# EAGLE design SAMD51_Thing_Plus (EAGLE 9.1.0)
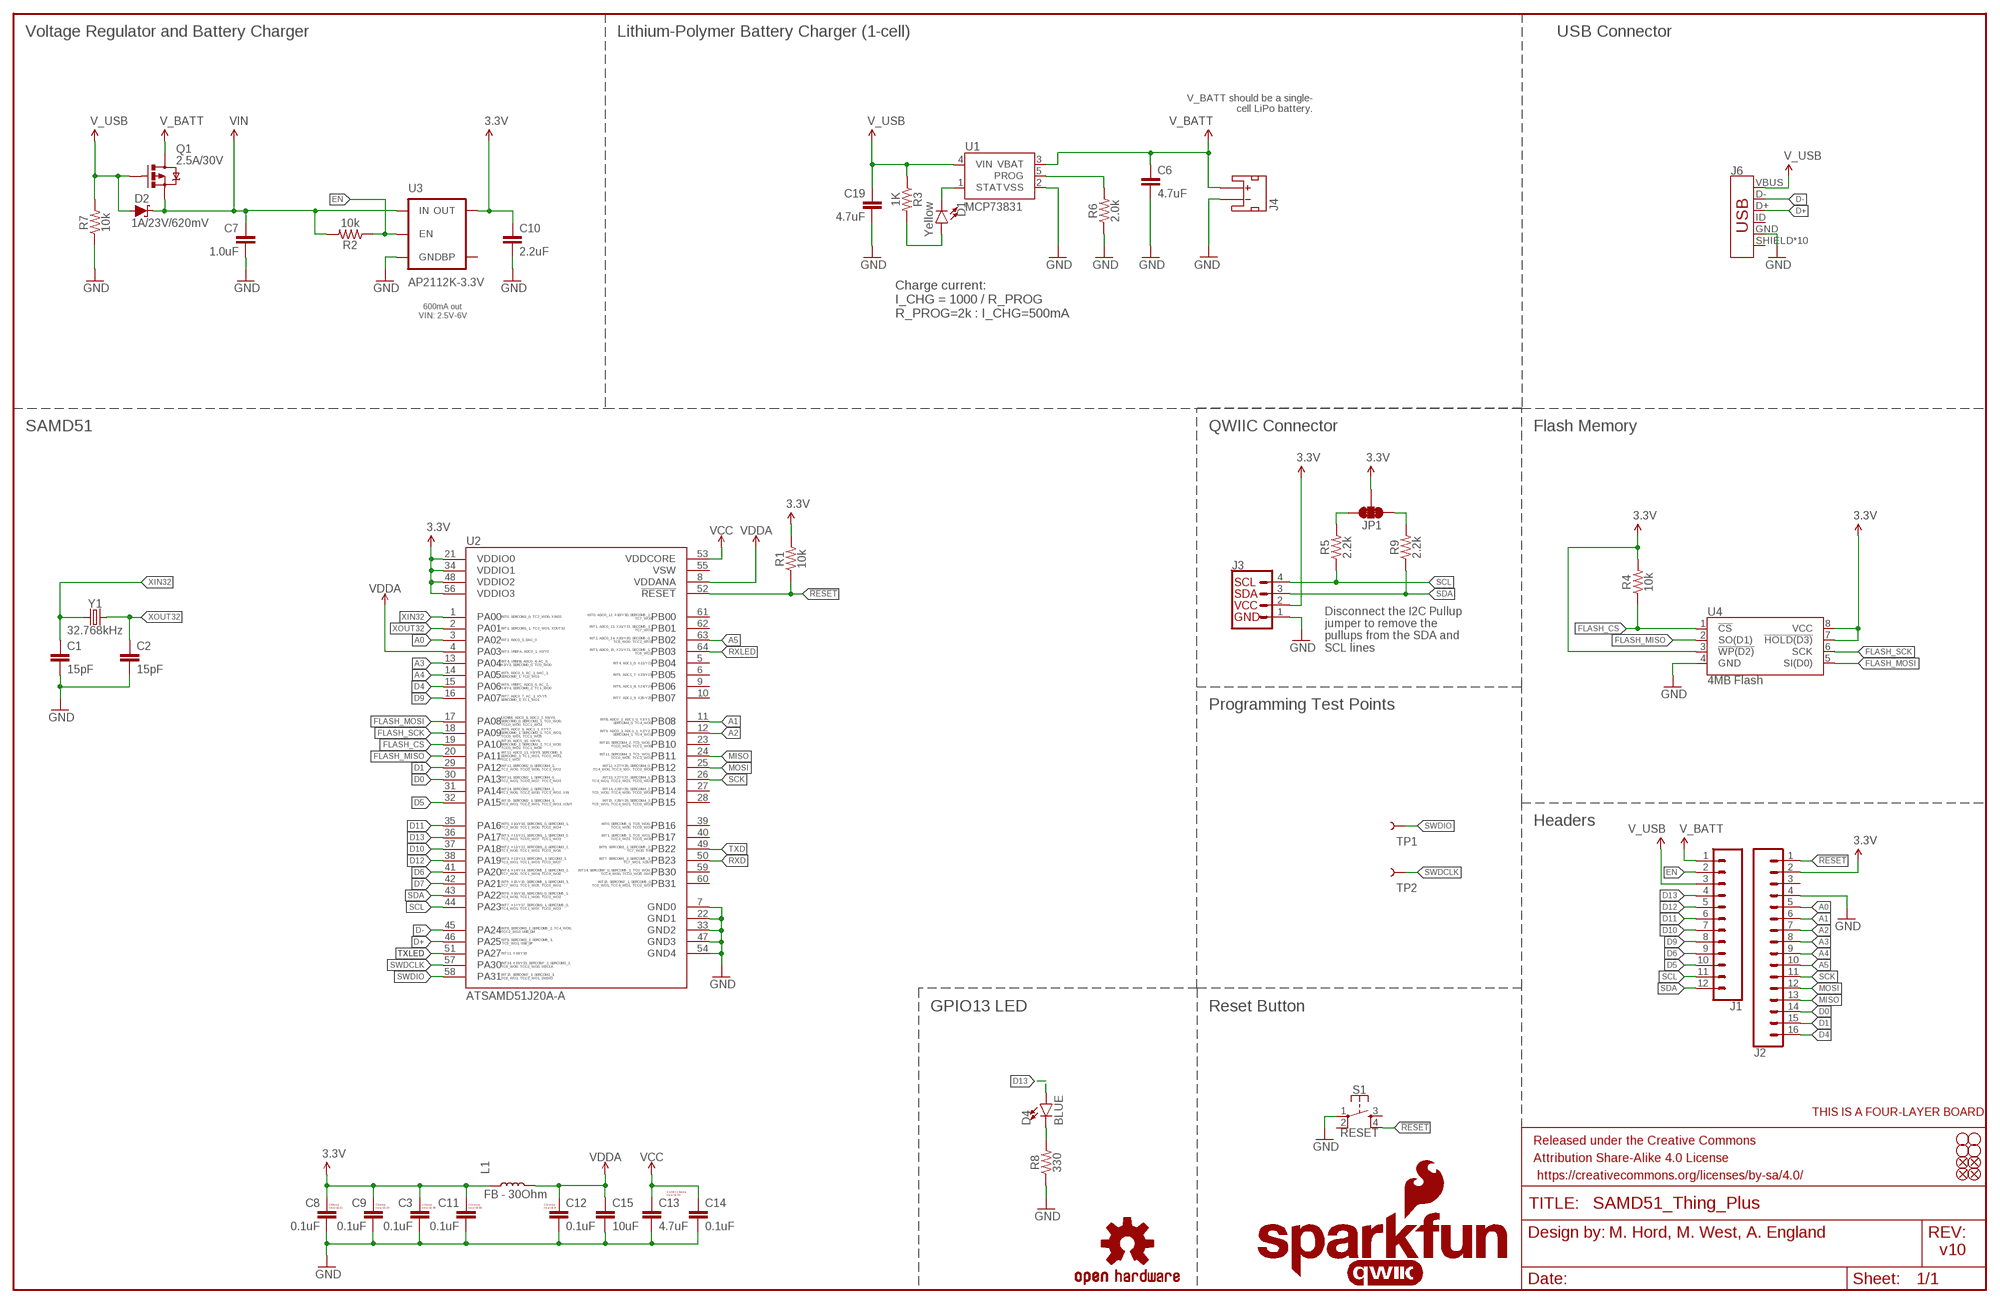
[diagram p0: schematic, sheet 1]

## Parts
C1  15pF  15PF-0402-50V-5%  [0402]
C2  15pF  15PF-0402-50V-5%  [0402]
C3  0.1uF  0.1UF-0402-16V-10%  [0402]
C6  4.7uF  4.7UF-0603-6.3V-(10%)  [0603]
C7  1.0uF  1.0UF-0603-16V-10%-X7R  [0603]
C8  0.1uF  0.1UF-0402-16V-10%  [0402]
C9  0.1uF  0.1UF-0402-16V-10%  [0402]
C10  2.2uF  2.2UF-0603-10V-20%  [0603]
C11  0.1uF  0.1UF-0402-16V-10%  [0402]
C12  0.1uF  0.1UF-0402-16V-10%  [0402]
C13  4.7uF  4.7UF-0603-6.3V-(10%)  [0603]
C14  0.1uF  0.1UF-0402-16V-10%  [0402]
C15  10uF  10UF-0805-10V-10%  [0805]
C19  4.7uF  4.7UF-0603-6.3V-(10%)  [0603]
D1  Yellow  LED-YELLOW0603  [LED-0603]
D2  1A/23V/620mV  DIODE-SCHOTTKY-BAT20J  [SOD-323]
D4  BLUE  LED-BLUE0603  [LED-0603]
FD1  FIDUCIALUFIDUCIAL  [FIDUCIAL-MICRO]
FD2  FIDUCIALUFIDUCIAL  [FIDUCIAL-MICRO]
FD3  FIDUCIALUFIDUCIAL  [FIDUCIAL-MICRO]
FD4  FIDUCIALUFIDUCIAL  [FIDUCIAL-MICRO]
FRAME1  FRAME-LEDGER  [CREATIVE_COMMONS]
H1  STAND-OFF  [STAND-OFF]
H2  STAND-OFF  [STAND-OFF]
H3  STAND-OFF  [STAND-OFF]
H4  STAND-OFF  [STAND-OFF]
J1  CONN_12SM_SQ_NO_SILK  [1X12_SM_SQ_NOSILK]
J2  CONN_161X16_SM_SQ_NOSILK  [1X16_SM_SQ_NOSILK]
J3  QWIIC_CONNECTORJS-1MM  [JST04_1MM_RA]
J4  JST_2MM_MALE  [JST-2-SMD]
J6  AMP FCI 10103594-0001LF  USB_MICRO-B_HALF_PTH_MILL  [USB-MICROB-PTH-MILL]
JP1  JUMPER-SMT_3_2-NC_TRACE_SILK  [SMT-JUMPER_3_2-NC_TRACE_SILK]
L1  FB - 30Ohm  INDUCTORFB-30OHM  [0603]
LOGO1  FOUR_LAYER_WARNING  [FOUR_LAYER_WARNING]
LOGO2  OSHW-LOGOMINI  [OSHW-LOGO-MINI]
LOGO3  SFE_LOGO_NAME_FLAME.1_INCH  [SFE_LOGO_NAME_FLAME_.1]
LOGO4  SFE_LOGO_FLAME.1_INCH  [SFE_LOGO_FLAME_.1]
Q1  2.5A/30V  MOSFET-PCHANNELDMG2307L  [SOT23-3@1]
R1  10k  10KOHM-0603-1/10W-1%  [0603]
R2  10k  10KOHM-0603-1/10W-1%  [0603]
R3  1K  1KOHM-1/10W-1%(0603)  [0603]
R4  10k  10KOHM-0603-1/10W-1%  [0603]
R5  2.2k  2.2KOHM-0603-1/10W-1%  [0603]
R6  2.0k  2.0KOHM1/10W5%(0603)  [0603]
R7  10k  10KOHM-0603-1/10W-1%  [0603]
R8  330  330OHM1/10W1%(0603)  [0603]
R9  2.2k  2.2KOHM-0603-1/10W-1%  [0603]
S1  RESET  MOMENTARY-SWITCH-SPST-2-SMD-4.6X2.8MM  [TACTILE_SWITCH_SMD_4.6X2.8MM]
TP1  TEST-POINTTP_15TH_THRU  [TP_15TH]
TP2  TEST-POINTTP_15TH_THRU  [TP_15TH]
U1  MCP73831  [SOT23-5]
U2  ATSAMD51J20A-A  [TQFP64]
U3  AP2112K-3.3V  V_REG_LDOSMD  [SOT23-5]
U4  4MB Flash  AT25SF041  [SO08]
U$69  QWIIC_LOGO_5MM  [QWIIC_5MM]
Y1  32.768kHz  CRYSTAL-32.768KHZSMD-3.2X1.5  [CRYSTAL-SMD-3.2X1.5MM]

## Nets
3.3V: C3.1 C8.1 C9.1 C10.1 C11.1 J2.2 J3.2 JP1.2 L1.1 R1.2 R4.2 U2.21(VDDIO0) U2.34(VDDIO1) U2.48(VDDIO2) U2.56(VDDIO3) U3.5(OUT) U4.3(!WP(D2)) U4.7(!HOLD(D3)) U4.8(VCC)
!RESET: J2.1 R1.1 S1.4 U2.52(!RESET)
A0: J2.5 U2.3(PA02)
A1: J2.6 U2.11(PB08)
A2: J2.7 U2.12(PB09)
A3: J2.8 U2.13(PA04)
A4: J2.9 U2.14(PA05)
A5: J2.10 U2.63(PB02)
D0: J2.14 U2.30(PA13)
D1: J2.15 U2.29(PA12)
D4: J2.16 U2.15(PA06)
D5: J1.10 U2.32(PA15)
D6: J1.9 U2.41(PA20)
D7: U2.42(PA21)
D9: J1.8 U2.16(PA07)
D10: J1.7 U2.37(PA18)
D11: J1.6 U2.35(PA16)
D12: J1.5 U2.38(PA19)
D13: D4.A J1.4 U2.36(PA17)
D+: J6.D+ U2.46(PA25)
D-: J6.D- U2.45(PA24)
EN: J1.2 R2.1 U3.3(EN)
FLASH_CS: R4.1 U2.19(PA10) U4.1(!CS)
FLASH_MISO: U2.20(PA11) U4.2(SO(D1))
FLASH_MOSI: U2.17(PA08) U4.5(SI(D0))
FLASH_SCK: U2.18(PA09) U4.6(SCK)
GND: C1.2 C2.2 C3.2 C6.2 C7.2 C8.2 C9.2 C10.2 C11.2 C12.2 C13.2 C14.2 C15.2 C19.2 J2.4 J3.1 J4.1(-) J6.GND R6.1 R7.1 R8.1 S1.1 U1.2(VSS) U2.7(GND0) U2.22(GND1) U2.33(GND2) U2.47(GND3) U2.54(GND4) U3.2(GND) U4.4(GND)
MISO: J2.13 U2.24(PB11)
MOSI: J2.12 U2.25(PB12)
N$1: D4.C R8.2
N$2: JP1.3 R5.2
N$3: JP1.1 R9.2
N$9: D1.C U1.1(STAT)
N$14: R6.2 U1.5(PROG)
N$17: D1.A R3.2
RXD: U2.50(PB23)
RXLED: U2.64(PB03)
SCK: J2.11 U2.26(PB13)
SCL: J1.11 J3.4 R5.1 U2.44(PA23)
SDA: J1.12 J3.3 R9.1 U2.43(PA22)
SWDCLK: TP2.P$1 U2.57(PA30)
SWDIO: TP1.P$1 U2.58(PA31)
TXD: U2.49(PB22)
TXLED: U2.51(PA27)
V_BATT: C6.1 J1.1 J4.2(+) Q1.3(D) U1.3(VBAT)
V_USB: C19.1 D2.A J1.3 J6.VBUS Q1.1(G) R3.1 R7.2 U1.4(VIN)
VCC: C13.1 C14.1 U2.53(VDDCORE)
VDDA: C12.1 C15.1 L1.2 U2.4(PA03) U2.8(VDDANA)
VIN: C7.1 D2.C Q1.2(S) R2.2 U3.1(IN)
XIN32: C1.1 U2.1(PA00) Y1.P$1
XOUT32: C2.1 U2.2(PA01) Y1.P$2
Unconnected: J2.3 J4.NC1(PAD1) J4.NC2(PAD2) J6.ID J6.SHIELD J6.SHIELD2(SHIELD) J6.SHIELD3(SHIELD) J6.SHIELD4(SHIELD) J6.SHIELD5(SHIELD) J6.SHIELD6(SHIELD) J6.SHIELD7(SHIELD) J6.SHIELD8(SHIELD) J6.SHIELD9(SHIELD) J6.SHIELD10(SHIELD) S1.2 S1.3 U2.5(PB04) U2.6(PB05) U2.9(PB06) U2.10(PB07) U2.23(PB10) U2.27(PB14) U2.28(PB15) U2.31(PA14) U2.39(PB16) U2.40(PB17) U2.55(VSW) U2.59(PB30) U2.60(PB31) U2.61(PB00) U2.62(PB01) U3.4(BP)

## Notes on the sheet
- Voltage Regulator and Battery Charger | Lithium-Polymer Battery Charger (1-cell)
- USB Connector
- V_BATT should be a single-
  cell LiPo battery.
- Charge current:
  I_CHG = 1000 / R_PROG
  R_PROG=2k : I_CHG=500mA
- 600mA out
  VIN: 2.5V-6V
- SAMD51 | QWIIC Connector | Flash Memory
- Disconnect the I2C Pullup 
  jumper to remove the 
  pullups from the SDA and 
  SCL lines
- Programming Test Points
- Headers
- GPIO13 LED | Reset Button
- C13 & C14 to be
  near U2.53
- C8 to be
  near U2.21
- C9 to be
  near U2.34
- C3 to be
  near U2.48
- C11 to be
  near U2.56
- C12 to be
  near U2.8
- M. Hord, M. West, A. England
- v10

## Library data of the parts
C1 C2 = SparkFun-Capacitors:15PF: 15pF ceramic capacitors; PROD_ID: CAP-13063
C3 C8 C9 C11 C12 C14 = SparkFun-Capacitors:0.1UF: 0.1µF ceramic capacitors; PROD_ID: CAP-12416
C6 C13 C19 = SparkFun-Capacitors:4.7UF: 4.7µF ceramic capacitors; PROD_ID: CAP-08280
C7 = SparkFun-Capacitors:1.0UF: 1µF ceramic capacitors; PROD_ID: CAP-13930
C10 = SparkFun-Capacitors:2.2UF: 2.2µF ceramic capacitors; PROD_ID: CAP-07888
C15 = SparkFun-Capacitors:10UF: 10.0µF ceramic capacitors; PROD_ID: CAP-11330
D1 = SparkFun-LED:LED-YELLOW: Yellow SMD LED; PROD_ID: DIO-09003
D2 = SparkFun-DiscreteSemi:DIODE-SCHOTTKY: Schottky diode; PROD_ID: DIO-11623
D4 = SparkFun-LED:LED-BLUE: Blue SMD LED; PROD_ID: DIO-08575
FD1-FD4 = SparkFun-Aesthetics:FIDUCIAL: Fiducial Alignment Points
FRAME1 = SparkFun-Aesthetics:FRAME-LEDGER: Schematic Frame - Ledger
H1-H4 = SparkFun-Hardware:STAND-OFF: Stand Off
J1 = SparkFun-Connectors:CONN_12: Multi connection point. Often used as Generic Header-pin footprint for 0.1 inch spaced/style header connections On any of the 0.1 inch spaced packages, you can populate with these: Break Away Headers - Straight (PRT-00116) Break Away Male Headers - Right Angle (PRT-00553) Female Headers (PRT-00115)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
J2 = SparkFun-Connectors:CONN_16: Multi connection point. Often used as Generic Header-pin footprint for 0.1 inch spaced/style header connections On any of the 0.1 inch spaced packages, you can populate with these: Break Away Headers - Straight (PRT-00116) Break Away Male Headers - Right Angle (PRT-00553) Female Headers (PRT-00115)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
J3 = SparkFun-Connectors:QWIIC_CONNECTOR: SparkFun I2C Standard Qwiic Connector An SMD 1mm pitch JST connector makes it easy and quick (get it? Qwiic?) to connect I2C devices to each other. The Qwiic system enables fast and solderless connection between popular platforms and various sensors and actuators. We carry 200mm, 100mm, 50mm, and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; PROD_ID: CONN-13694
J4 = SparkFun-Connectors:JST_2MM_MALE: JST 2MM MALE RA CONNECTOR Two pin, compact surface mount connector. Commonly used as a battery input connection point. We really like the solid locking feeling and high current rating on these small connectors. We use these all the time as battery connectors. Mates to single-cell LiPo batteries.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; PROD_ID: CONN-11443; SF_ID: PRT-08612
J6 = SparkFun-Connectors:USB_MICRO-B: USB Type Micro-B Connector Male/female and PTH/SMT variants SparkFun Products: SparkFun microB USB Breakout SparkFun USB microB Plug Breakout SparkFun ESP8266 Thing; PROD_ID: CONN-13711
JP1 = SparkFun-Jumpers:JUMPER-SMT_3_2-NC_TRACE: Normally closed trace jumper (2 of 2 connections) This jumper has a trace between all three pads so they are normally closed (NC). Use a razor knife to open the connection(s). For best results follow the IPC guidelines for cutting traces: Cutout at least 0.063 mm (0.005 in). Remove all loose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
L1 = SparkFun-Coils:INDUCTOR: Inductors; PROD_ID: NDUC-07859
LOGO1 = SparkFun-Aesthetics:FOUR_LAYER_WARNING: Four-Layer Board Warning - tDoc Layer
LOGO2 = SparkFun-Aesthetics:OSHW-LOGO: Open-Source Hardware (OSHW) Logo
LOGO3 = SparkFun-Aesthetics:SFE_LOGO_NAME_FLAME: SparkFun Font Logo w/ Flame
LOGO4 = SparkFun-Aesthetics:SFE_LOGO_FLAME: SparkFun Flame Logo
Q1 = SparkFun-DiscreteSemi:MOSFET-PCHANNEL: Generic PMOSFET IRLML2244 - TRANS-11153 (SOT-23 -20V -4.3A) (1.Gate 2.Source 3.Drain) FQP27P06 - COM-10349 (TO-220 -60V -27A) (1.Gate 2.Source 3.Drain); PROD_ID: TRANS-11308
R1 R2 R4 R7 = SparkFun-Resistors:10KOHM: 10kΩ resistor; PROD_ID: RES-00824
R3 = SparkFun-Resistors:1KOHM-1/10W-1%(0603): RES-07856; PROD_ID: RES-07856
R5 R9 = SparkFun-Resistors:2.2KOHM: 2.2kΩ resistor; PROD_ID: RES-08272
R6 = SparkFun-Resistors:2.0KOHM1/10W5%(0603): RES-08296; PROD_ID: RES-08296
R8 = SparkFun-Resistors:330OHM1/10W1%(0603): RES-00818; PROD_ID: RES-00818
S1 = SparkFun-Switches:MOMENTARY-SWITCH-SPST-2: Momentary Switch (Pushbutton) - SPST - Two Circuits Normally-open (NO) SPST momentary switches (buttons, pushbuttons). Schematic symbol includes two switch circuits. Variants SMD-4.6MMX2.8MM - 4.60mm x 2.80mm Tactile Momentary Button Switch - Used on SparkFun SAMD21 Mini Breakout SMD-5.2MM - Mini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; PROD_ID: SWCH-13065
TP1 TP2 = SparkFun-Connectors:TEST-POINT: SparkFun Test Points
U1 = SparkFun-PowerIC:MCP73831: Miniature single cell, fully integrated Li-Ion, Li-polymer charge management controller http://ww1.microchip.com/downloads/en/DeviceDoc/20001984g.pdf IC-09995; PROD_ID: IC-09995
U2 = SparkFun-IC-Microcontroller:ATSAMD51J20A-A; PROD_ID: IC-13952
U3 = SparkFun-PowerIC:V_REG_LDO: Voltage Regulator LDO Standard 150mA LDO voltage regulator in SOT-23 layout. Micrel part MIC5205. BP (by-pass) pin is used to lower output noise with 470pF cap.; PROD_ID: VREG-12457
U4 = SparkFun-IC-Memory:AT25SF041: AT25SF041 4Mb Serial Flash Memory 104MHz, SPI, 8-SOIC Datasheet SparkFun Products: SparkFun ESP8266 Thing SparkFun ESP8266 Thing - Dev Board; PROD_ID: IC-12455
U$69 = SparkFun-Aesthetics:QWIIC_LOGO: Qwiic Logos for placement on schematic and PCB. The 5.5mm silk logo is best for placing next to Qwiic connector.
Y1 = SparkFun-Clocks:CRYSTAL-32.768KHZ: 32.768kHz Crystal; PROD_ID: XTAL-13062

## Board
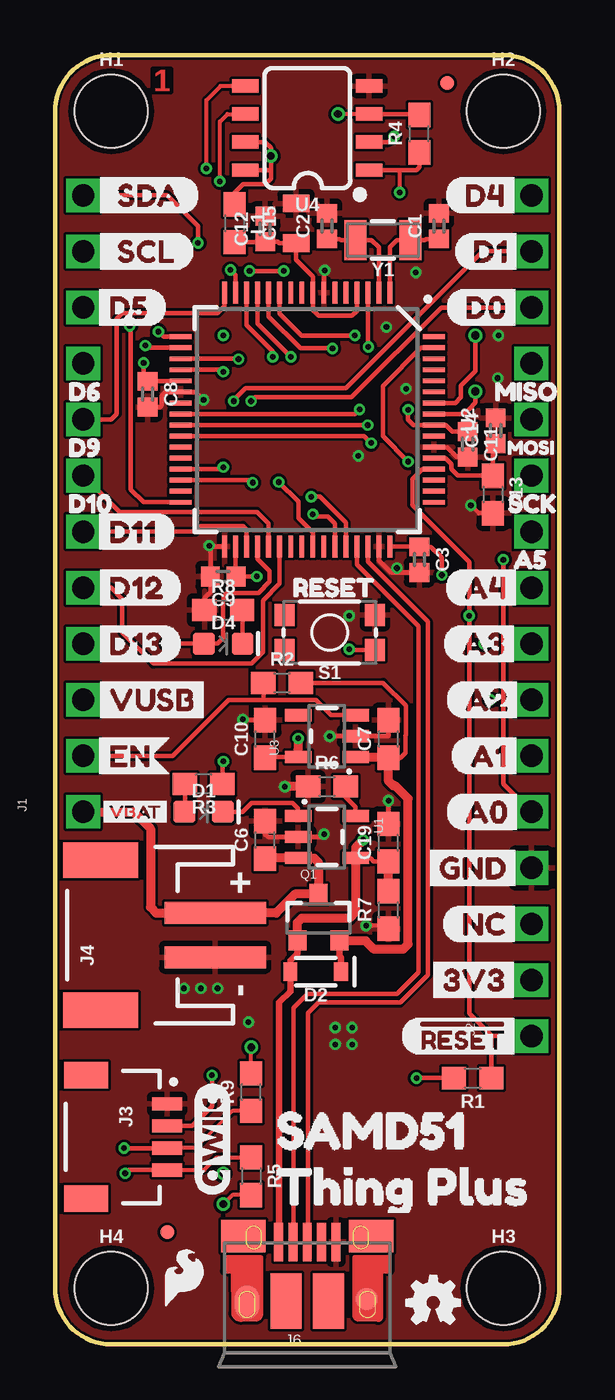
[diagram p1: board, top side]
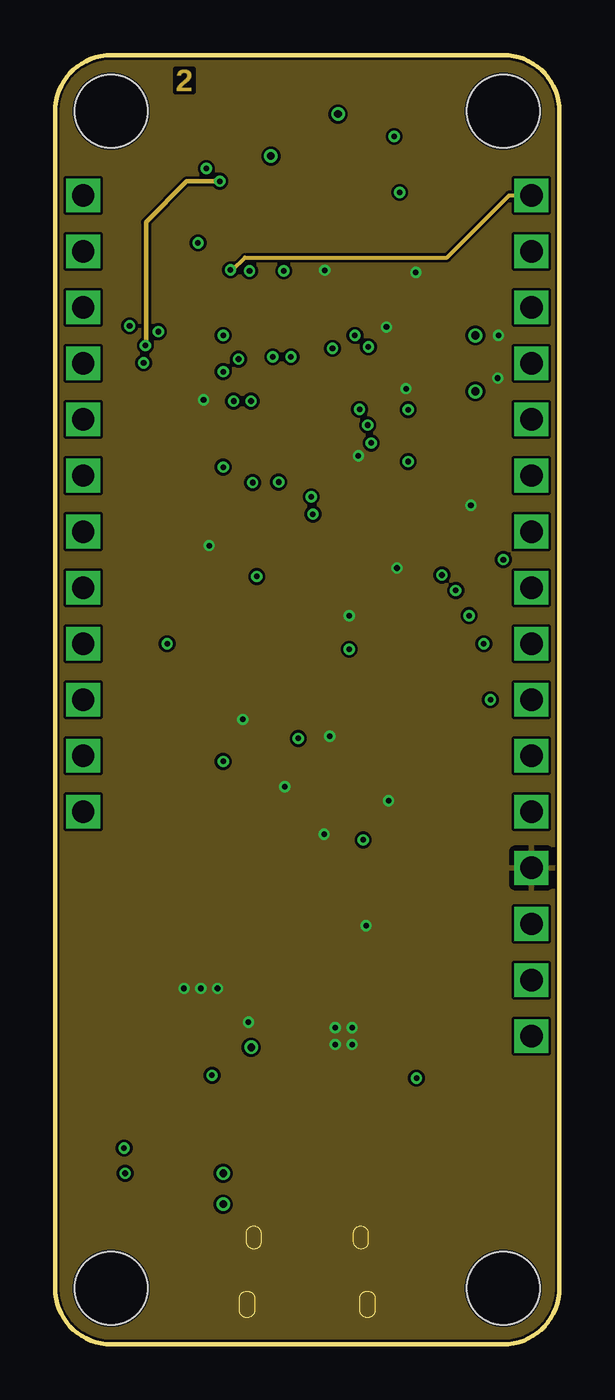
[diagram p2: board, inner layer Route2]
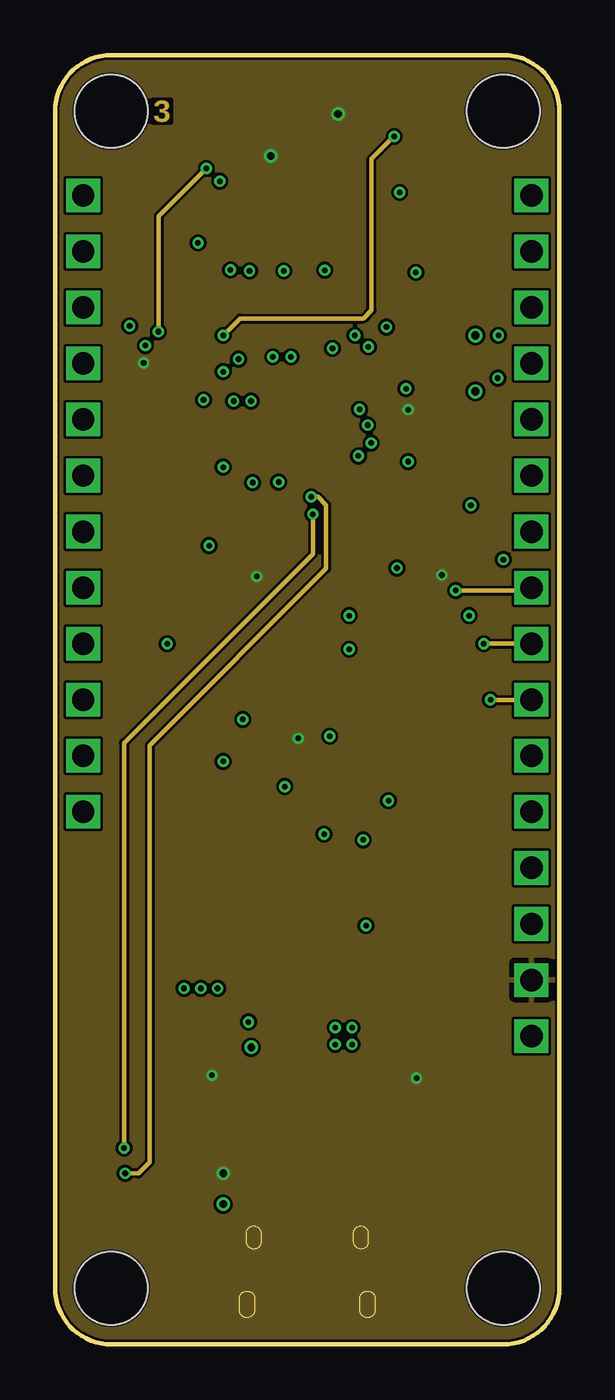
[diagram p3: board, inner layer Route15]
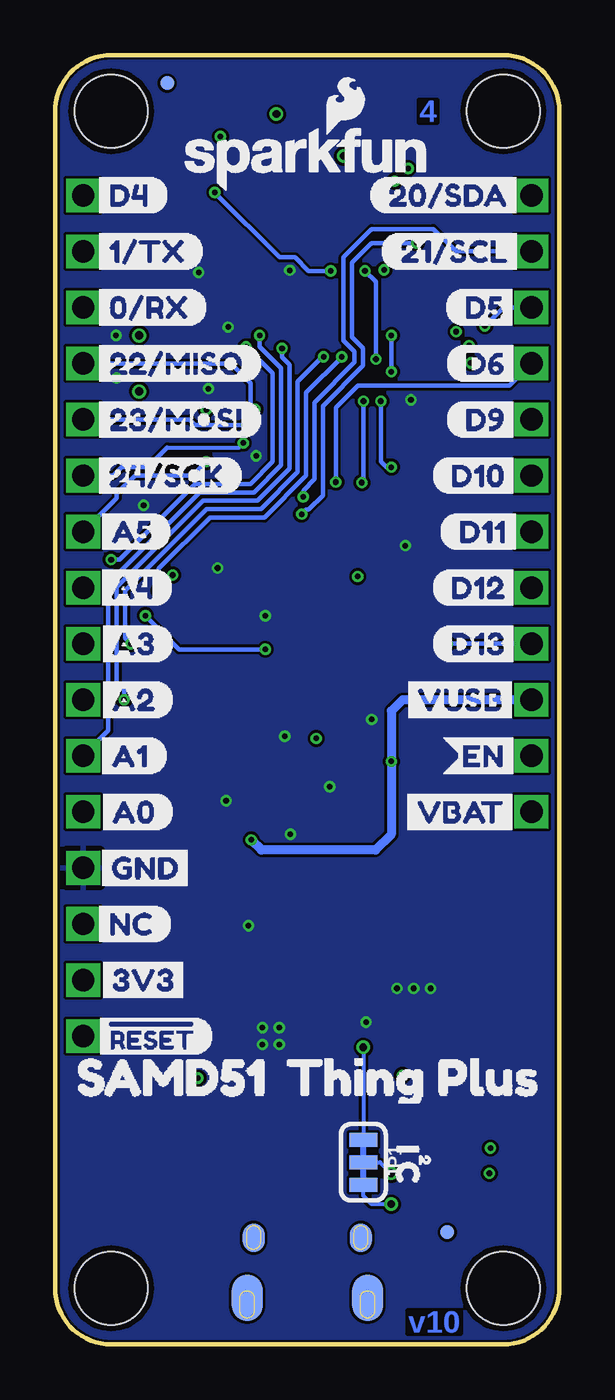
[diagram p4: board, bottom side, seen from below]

Size 22.86 x 58.42 mm. Coordinates in mm from the lower left corner, seen from the top.
Outline: 2.54,58.42 20.32,58.42 arc-90 22.86,55.88 22.86,2.54 arc-90 20.32,0 2.54,0 arc-90 0,2.54 0,55.88 arc-90 2.54,58.42
Copper layers (1*2*15*16): Top 0.035559375mm / dielectric 0.47751875mm / Route2 0.035559375mm / dielectric 0.47751875mm / Route15 0.035559375mm / dielectric 0.47751875mm / Bottom 0.035559375mm
Design rules "SparkFun-4-layer-FAB-LIMIT": minimum track width 4mil, minimum drill 6mil, track to track 5mil, track to pad 5mil, pad to pad 5mil, via to via 5mil, smd to smd 5mil, copper to edge 4mil, drill to drill 4mil, minimum pad ring 5mil, minimum via ring 5mil, stop-mask expansion 4mil, vias tented up to drill 25mil, thermal gap 10mil

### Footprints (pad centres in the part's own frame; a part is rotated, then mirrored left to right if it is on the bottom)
0402 = smd 0.85 x 0.9: 1 -0.58,0; 2 0.58,0
0603 = smd 1.1 x 1: 1 -0.85,0; 2 0.85,0
0805 = smd 0.8 x 1.2: 1 -0.9,0; 2 0.9,0
LED-0603 = smd 1 x 1: A -0.877,0; C 0.877,0
SOD-323 = smd 0.63 x 0.83: A 1.15,0; C -1.15,0
FIDUCIAL-MICRO = smd 0.635 x 0.635: 1 0,0
STAND-OFF = hole 3.302: 0,0
1X12_SM_SQ_NOSILK = drill 1.016 pad 1.27 square: 1 0,0; 2 2.54,0; 3 5.08,0; 4 7.62,0; 5 10.16,0; 6 12.7,0; 7 15.24,0; 8 17.78,0; 9 20.32,0; 10 22.86,0; 11 25.4,0; 12 27.94,0
1X16_SM_SQ_NOSILK = drill 1.016 pad 1.27 square: 1 0,0; 2 2.54,0; 3 5.08,0; 4 7.62,0; 5 10.16,0; 6 12.7,0; 7 15.24,0; 8 17.78,0; 9 20.32,0; 10 22.86,0; 11 25.4,0; 12 27.94,0; 13 30.48,0; 14 33.02,0; 15 35.56,0; 16 38.1,0
JST04_1MM_RA = smd 0.6 x 1.35: 1 -1.5,0; 2 -0.5,0; 3 0.5,0; 4 1.5,0 | smd 1.2 x 2: NC1 2.8,-3.675; NC2 -2.8,-3.675
JST-2-SMD = smd 1 x 4.6: 1 -1,-3.7; 2 1,-3.7 | smd 1.6 x 3.4: NC1 -3.4,1.5; NC2 3.4,1.5
USB-MICROB-PTH-MILL = smd 0.4 x 1.75: D+ 0,0; D- -0.65,0; GND 1.3,0; ID 0.65,0; VBUS -1.3,0 | smd 2 x 1.46: SHIELD -2.9,0.275; SHIELD2 2.9,0.275 | smd 1.425 x 2.5: SHIELD3 -0.963,-2.675; SHIELD4 0.963,-2.675 | smd 1.4 x 2.1 bottom: SHIELD5 -2.731,-2.531; SHIELD7 2.729,-2.531 | smd 1 x 1: SHIELD6 2.7,-2.575 | smd 1.1 x 1.5: SHIELD8 -2.731,-2.731 | smd 1 x 1.3 bottom: SHIELD9 -2.43,0.195; SHIELD10 2.43,0.195
SMT-JUMPER_3_2-NC_TRACE_SILK = smd 0.635 x 1.27: 1 -1.016,0; 2 0,0; 3 1.016,0
SOT23-3@1 = smd 0.8 x 0.9: 1 -0.95,-1; 2 0.95,-1; 3 0,1.1
TACTILE_SWITCH_SMD_4.6X2.8MM = smd 0.9 x 1: 1 -2.05,-0.8; 2 2.05,-0.8; 3 2.05,0.8; 4 -2.05,0.8
TP_15TH = drill 0.381 pad 0.61: P$1 0,0
SOT23-5 = smd 0.55 x 1.2: 1 -0.95,-1.3; 2 0,-1.3; 3 0.95,-1.3; 4 0.95,1.3; 5 -0.95,1.3
TQFP64 = smd 0.22 x 1: 1 -3.75,-5.75; 2 -3.25,-5.75; 3 -2.75,-5.75; 4 -2.25,-5.75; 5 -1.75,-5.75; 6 -1.25,-5.75; 7 -0.75,-5.75; 8 -0.25,-5.75; 9 0.25,-5.75; 10 0.75,-5.75; 11 1.25,-5.75; 12 1.75,-5.75; 13 2.25,-5.75; 14 2.75,-5.75; 15 3.25,-5.75; 16 3.75,-5.75; 33 3.75,5.75; 34 3.25,5.75; 35 2.75,5.75; 36 2.25,5.75; 37 1.75,5.75; 38 1.25,5.75; 39 0.75,5.75; 40 0.25,5.75; 41 -0.25,5.75; 42 -0.75,5.75; 43 -1.25,5.75; 44 -1.75,5.75; 45 -2.25,5.75; 46 -2.75,5.75; 47 -3.25,5.75; 48 -3.75,5.75 | smd 1 x 0.22: 17 5.75,-3.75; 18 5.75,-3.25; 19 5.75,-2.75; 20 5.75,-2.25; 21 5.75,-1.75; 22 5.75,-1.25; 23 5.75,-0.75; 24 5.75,-0.25; 25 5.75,0.25; 26 5.75,0.75; 27 5.75,1.25; 28 5.75,1.75; 29 5.75,2.25; 30 5.75,2.75; 31 5.75,3.25; 32 5.75,3.75; 49 -5.75,3.75; 50 -5.75,3.25; 51 -5.75,2.75; 52 -5.75,2.25; 53 -5.75,1.75; 54 -5.75,1.25; 55 -5.75,0.75; 56 -5.75,0.25; 57 -5.75,-0.25; 58 -5.75,-0.75; 59 -5.75,-1.25; 60 -5.75,-1.75; 61 -5.75,-2.25; 62 -5.75,-2.75; 63 -5.75,-3.25; 64 -5.75,-3.75
SO08 = smd 0.6 x 1.2: 1 -1.905,-2.8; 2 -0.635,-2.8; 3 0.635,-2.8; 4 1.905,-2.8; 5 1.905,2.8; 6 0.635,2.8; 7 -0.635,2.8; 8 -1.905,2.8
CRYSTAL-SMD-3.2X1.5MM = smd 1 x 1.8: P$1 -1.25,0; P$2 1.25,0

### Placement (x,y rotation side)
C1  17.4,50.67 90 top
C2  12.32,50.67 90 top
C3  16.51,35.56 270 top
C6  9.53,22.86 90 top
C7  15.11,27.43 90 top
C8  4.19,43.05 270 top
C9  7.62,34.8 180 top
C10  9.53,27.43 90 top
C11  18.7,40.79 270 top
C12  9.53,50.55 90 top
C13  19.84,38.51 270 top
C14  19.97,41.4 90 top
C15  10.92,50.8 90 top
C19  15.11,22.73 90 top
D1  6.73,24.13 0 top
D2  11.81,16.89 180 top
D4  7.62,31.75 0 top
FD1  5.08,5.08 0 top
FD2  17.78,57.15 0 top
FD3  5.08,5.08 0 bottom
FD4  17.78,57.15 0 bottom
FRAME1  not placed on the board
H1  2.54,55.88 0 top
H2  20.32,55.88 0 top
H3  20.32,2.54 0 top
H4  2.54,2.54 0 top
J1  1.27,24.13 90 top
J2  21.59,13.97 90 top
J3  5.08,9.4 270 top
J4  3.56,18.54 90 top
J6  11.43,4.64 0 top
JP1  8.89,8.26 270 bottom
L1  8.13,50.8 270 top
LOGO1  not placed on the board
LOGO2  17.14,1.91 0 top
LOGO3  11.43,53.72 0 bottom
LOGO4  5.84,3.05 0 top
Q1  11.94,19.3 0 top
R1  18.92,12.06 180 top
R2  10.29,29.97 0 top
R3  6.73,25.4 180 top
R4  16.51,54.86 90 top
R5  8.89,7.62 270 top
R6  12.32,25.27 0 top
R7  15.11,19.68 90 top
R8  7.62,33.27 0 top
R9  8.89,11.43 90 top
S1  12.45,32.26 180 top
TP1  19.05,45.72 0 top
TP2  19.05,43.18 0 top
U1  12.32,22.99 270 top
U2  11.43,41.91 180 top
U3  12.32,27.56 90 top
U4  11.43,55.12 90 top
U$4  [RESET27]  10.03,34.29 0 top
U$5  [#RESET15]  21.46,13.97 0 bottom
U$6  [#RESET0]  15.49,13.97 0 top
U$7  [3V32]  16.64,16.51 0 top
U$8  [A04]  17.65,24.13 0 top
U$9  [A15]  17.91,26.67 0 top
U$10  [A26]  17.65,29.21 0 top
U$11  [A37]  17.53,31.75 0 top
U$12  [A48]  17.65,34.29 0 top
U$13  [A523]  20.07,35.56 0 top
U$14  [SCK24]  19.81,38.1 0 top
U$15  [3V33]  21.21,16.51 0 bottom
U$16  [MISO26]  19.18,43.18 0 top
U$17  [D09]  17.65,46.99 0 top
U$18  [D110]  18.03,49.53 0 top
U$19  [D411]  17.65,52.07 0 top
U$20  [GND3]  16.51,21.59 0 top
U$21  [GND0]  21.21,21.59 0 bottom
U$22  [EN0]  1.52,26.67 0 top
U$23  [VUSB2]  1.52,29.21 0 top
U$24  [D1312]  1.52,31.75 0 top
U$25  [D120]  1.52,34.29 0 top
U$26  [D1113]  1.52,36.83 0 top
U$27  [A014]  21.21,24.13 0 bottom
U$28  [A113]  21.21,26.67 0 bottom
U$29  [D515]  1.52,46.99 0 top
U$30  [_SCL16]  1.52,49.53 0 top
U$31  [ORDERING_INSTRUCTIONS]  not placed on the board
U$32  [_SDA17]  1.52,52.07 0 top
U$33  [D63]  -0.13,43.18 0 top
U$34  [D92]  -0.13,40.64 0 top
U$35  [MOSI0]  19.94,40.64 0 top
U$36  [VBAT1]  1.91,24.13 0 top
U$37  [A212]  21.21,29.21 0 bottom
U$38  [A311]  21.21,31.75 0 bottom
U$39  [A410]  21.21,34.29 0 bottom
U$40  [A59]  21.21,36.83 0 bottom
U$41  [21#SCL1]  8.13,49.53 0 bottom
U$42  [22#MISO4]  21.34,44.45 0 bottom
U$43  [23#MOSI3]  21.34,41.91 0 bottom
U$44  [1#TX1]  21.34,49.53 0 bottom
U$46  [D41]  21.34,52.07 0 bottom
U$47  [24#SCK2]  21.34,39.37 0 bottom
U$48  [0#RX0]  21.34,46.99 0 bottom
U$49  [D518]  5.21,46.99 0 bottom
U$50  [D619]  5.21,44.45 0 bottom
U$51  [D920]  5.21,41.91 0 bottom
U$52  [D1122]  5.46,36.83 0 bottom
U$53  [D1021]  5.84,39.37 0 bottom
U$54  [D1223]  5.84,34.29 0 bottom
U$55  [D1324]  5.84,31.75 0 bottom
U$56  [VUSB1]  7.37,29.21 0 bottom
U$57  [EN25]  5.33,26.67 0 bottom
U$58  [VBAT2]  7.37,24.13 0 bottom
U$59  [D100]  -0.13,38.1 0 top
U$60  [NC0]  17.53,19.05 0 top
U$61  [NC1]  21.34,19.05 0 bottom
U$62  [20#SDA0]  8.64,52.07 0 bottom
U$63  [SAMD510]  8.89,9.53 0 top
U$64  [THING_PLUS1]  8.89,6.99 0 top
U$65  [SAMD510]  23.02,11.94 0 bottom
U$66  [THING_PLUS1]  13.49,11.94 0 bottom
U$67  [I_C0]  6.86,9.91 270 bottom
U$68  [21]  6.1,9.02 270 bottom
U$69  7.11,9.27 90 top
Y1  14.86,50.04 180 top

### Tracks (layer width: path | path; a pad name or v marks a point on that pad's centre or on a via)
3.3V  (via drill 0.25, 0.35)
  Top 0.178: U4.3 12.89,55.75 v12.83,55.75
  Top 0.203: U2.48 16.49,36.16 C3.1 17.04,36.14 17.53,35.65 v17.53,34.86 | U2.34 8.18,34.82 C9.1 v9.14,34.8 | U2.21 4.22,43.66 C8.1 4.01,43.81 v4.01,44.48 | U3.5 9.55,26.61 C10.1 | R1.2 v16.38,12.06 | U4.3 16.47,55.75 R4.2 | C11.1 18.01,41.37 17.71,41.66 U2.56 16.25,41.66 16,41.91 v16,42.35 | L1.1 8.13,52.2 8.51,52.58 9.53,52.58 9.78,52.83 9.78,53.21 | U4.7 9.53,54.48 9.78,54.23 v9.78,53.85 9.78,53.21 | U4.8 9.78,53.21 | v7.11,12.19 7.11,10.79 6.21,9.9 J3.2
  Top 0.406: U3.5 11.02,26.99 v11.02,27.46
  Bottom 0.178: JP1.2 8.13,8.26 v7.62,7.75
  pour Route15: 0,58.42 22.86,58.42 22.86,0 0,0
!RESET  (via drill 0.25)
  Top 0.203: S1.4 13.37,31.46 | U2.52 16.64,39.66 16.19,39.21 16.19,38.1 16.19,38.04 18.77,35.46 v18.77,33.02 18.77,15 19.77,14 19.77,13.97 | 19.77,13.97 R1.1 | J2.1 19.77,13.97
  Top 0.254: 13.37,31.46 v13.34,31.5
  Bottom 0.203: v13.34,31.5 17.25,31.5 v18.77,33.02
A0  (via drill 0.25)
  Top 0.203: v20.32,35.56 20.32,25.4 J2.5 | U2.3 14.18,45.22 v14.2,45.2
  Bottom 0.203: 13.01,44.01 13.01,39.99 14.01,38.99 16.51,38.99 19.94,35.56 v20.32,35.56 | 13.01,44.01 | 13.01,44.01 v14.2,45.2
A1  (via drill 0.25)
  Top 0.203: U2.11 10.18,46.72 11.18,45.72 v13.59,45.72
  Bottom 0.203: v13.59,45.72 13.59,45.21 12.62,44.25 12.62,39.83 13.85,38.61 16.32,38.61 20.45,34.48 20.45,27.81 J2.6
A2  (via drill 0.25)
  Top 0.203: U2.12 9.68,46.58 11.12,45.14 v12.57,45.14
  Route15 0.203: v19.74,29.21 J2.7
  Bottom 0.203: v12.57,45.14 12.57,44.74 12.24,44.41 12.24,39.68 13.69,38.23 16.16,38.23 20.07,34.32 20.07,29.97 19.74,29.64 v19.74,29.21
A3  (via drill 0.25)
  Top 0.203: U2.13 9.18,46.26 v10.69,44.74
  Route15 0.203: v19.43,31.75 J2.8
  Bottom 0.203: v10.69,44.74 10.76,44.74 11.86,43.64 11.86,39.52 13.53,37.85 16,37.85 19.68,34.16 19.68,32 v19.43,31.75
A4  (via drill 0.25)
  Top 0.203: U2.14 8.68,46.18 9.86,45 v9.86,44.74
  Route15 0.203: v18.16,34.16 21.46,34.16 J2.9
  Bottom 0.203: v9.86,44.74 11.48,43.13 11.48,39.36 13.38,37.47 15.85,37.47 18.16,35.15 v18.16,34.16
A5  (via drill 0.25)
  Top 0.203: U2.63 16.59,45.16 14.86,43.43 14.86,41.15 v16,40.01
  Bottom 0.203: v16,40.01 16.64,39.37 19.24,39.37 20.07,38.54 20.07,38.35 J2.10
D0  (via drill 0.25)
  Top 0.203: J2.14 17.5,46.99 13.44,42.93 9.06,42.93 v8.88,42.74 | v8.95,39.05 8.84,39.16 U2.30
  Bottom 0.203: v8.88,42.74 8.88,39.12 v8.95,39.05
D1  (via drill 0.25)
  Top 0.203: v8.09,42.74 8.09,42.78 8.64,43.33 13.19,43.33 19.39,49.53 J2.15 | v7.62,39.75 7.53,39.66 U2.29
  Bottom 0.203: v8.09,42.74 8.09,40.01 7.84,39.75 v7.62,39.75
D4  (via drill 0.25)
  Top 0.203: U2.15 8.18,48.46 v7.95,48.69
  Route2 0.178: v7.95,48.69 8.05,48.69 8.61,49.24 17.76,49.24 20.59,52.07 J2.16
D5  (via drill 0.25)
  Top 0.203: U2.32 4,38.16 3.43,38.73 3.43,44.45 3.43,46.1 v3.38,46.15
  Bottom 0.203: v3.38,46.15 2.54,46.99 J1.10
D6  (via drill 0.25)
  Top 0.203: v10.13,39.08 11.03,38.19 11.03,37.45 11.68,36.8 U2.41
  Bottom 0.203: v10.13,39.08 10.13,42.44 9.12,43.45 2.27,43.45 J1.9
D9
  Top 0.203: U2.16 7.68,47.05 7.37,46.74 3.05,46.74 2.79,46.48 2.79,42.16 2.54,41.91 J1.8
D10
  Top 0.203: U2.37 9.68,37.18 9.14,37.72 2.92,37.72 J1.7
D11
  Top 0.203: U2.35 8.68,36.91 8.51,37.08 6.6,37.08 6.35,36.83 J1.6
D12
  Top 0.203: J1.5 2.54,34.29 3.05,33.78 3.05,32.26 4.46,30.84 8.9,30.84 9.43,31.37 9.43,33.72 10.18,34.47 U2.38
D13  (via drill 0.25)
  Top 0.203: U2.36 9.18,35.59 9.73,35.04 9.73,34.56 9.23,34.05 7.8,34.05 7.64,33.89 7.64,33.68 7.62,33.66 7.62,32 7.37,31.75 D4.A 5.46,31.75 v5.08,31.75
  Bottom 0.203: v5.08,31.75 J1.4
D+
  Top 0.203: J6.D+ 11.46,4.66 11.46,15.01 11.94,15.49 15.65,15.49 16.89,16.73 16.89,32.77 14.18,35.48 U2.46
D-
  Top 0.203: U2.45 13.68,35.34 14.61,34.42 16.48,32.55 16.48,16.86 15.49,15.88 11.43,15.88 10.81,15.25 10.81,4.66 J6.D-
EN
  Top 0.203: J1.2 5.33,26.67 7.86,29.19 9.4,29.19 | U3.3 12.51,28.51 11.83,29.19 9.4,29.19 | R2.1 9.44,29.23 9.4,29.19
FLASH_CS  (via drill 0.25)
  Top 0.178: v15.62,52.2 15.62,53.15 15.56,53.21
  Top 0.203: 15.56,53.21 15.24,53.21 | 15.24,53.21 U4.1 | v10.36,48.64 v8.81,48.64 | U2.19 8.3,44.66 v8.31,44.64 | 15.24,53.21 16.38,53.21 16.51,53.34 R4.1
  Bottom 0.203: v15.62,52.2 12.68,49.26 11.98,49.26 11.37,48.64 v10.36,48.64 | v8.81,48.64 8.31,48.15 v8.31,44.64
FLASH_MISO  (via drill 0.25)
  Top 0.203: 7.54,44.16 v7.62,44.08 7.54,44.16 | U4.2 15.11,54.48 v15.37,54.74 | 7.54,44.16 U2.20
  Route15 0.203: v7.62,45.72 8.38,46.48 13.97,46.48 14.35,46.86 14.35,53.72 v15.37,54.74
  Bottom 0.203: v7.62,44.08 v7.62,45.72
FLASH_MOSI  (via drill 0.25)
  Top 0.178: U4.5 7.49,57.02 6.86,56.39 v6.86,53.29
  Top 0.203: v4.68,45.89 4.91,45.66 U2.17
  Route15 0.203: v6.86,53.29 4.7,51.13 4.7,45.91 v4.68,45.89
FLASH_SCK  (via drill 0.25)
  Top 0.178: v7.47,52.7 7.47,55.41 7.81,55.75 U4.6
  Top 0.203: U2.18 4.19,45.16 v4.09,45.26
  Route2 0.203: v7.47,52.7 5.97,52.7 4.12,50.85 4.12,45.24 v4.09,45.26
GND  (via drill 0.25)
  Top 0.178: C13.2 19.21,37.66 v18.85,38.02
  Top 0.203: C6.2 9.53,23.11 9.65,22.99 U1.2 12.06,22.99 v12.19,23.11 | C19.2 v15.11,24.64 | v12.45,27.56 U3.2 15.11,27.56 C7.2 | C10.2 8.55,28.28 v8.51,28.32 | R8.1 6.77,33.82 7.04,34.09 C9.2 7.04,36.14 v6.99,36.2 7.02,36.16 U2.33 | R7.1 14.97,18.97 v14.1,18.97 | v6.73,42.8 6.37,43.16 U2.22 4.99,43.16 4.83,43 4.83,42.55 4.75,42.47 C8.2 | U2.7 12.18,48.63 v12.22,48.67 | U2.54 17.2,40.64 17.78,40.64 18.21,40.21 C11.2 | U2.47 14.68,35.52 15.22,34.98 C3.2
  Top 0.406: R6.1 v10.41,25.27
  other vias: 20.07,43.78 15.49,35.18 13.34,33.02 12.7,13.59 12.7,14.35 13.46,14.35 13.46,13.59 5.84,16.13 6.6,16.13 7.37,16.13 8.76,14.61 16.35,48.58 13.75,40.26 20.1,45.72 15.02,46.1 15.91,43.31
  pour Top: 0,58.42 22.86,58.42 22.86,0 0,0
  pour Route2: 0,58.42 22.86,58.42 22.86,0 0,0
  pour Bottom: 0,58.42 22.86,58.42 22.86,0 0,0
MISO  (via drill 0.25)
  Top 0.203: U2.24 13.59,42.16 v13.8,42.37
  Bottom 0.203: v13.8,42.37 14,42.57 14,43.57 14.88,44.45 J2.13
MOSI  (via drill 0.25)
  Top 0.203: U2.25 v14.17,41.66
  Bottom 0.203: J2.12 16.76,41.91 16.51,41.66 v14.17,41.66
N$1
  Top 0.203: R8.2 8.5,33.25 D4.C
N$2  (via drill 0.35)
  Top 0.178: R5.2 8.04,6.77 v7.62,6.35
  Bottom 0.178: v7.62,6.35 8.51,6.35 8.89,6.73 JP1.3
N$3  (via drill 0.35)
  Top 0.178: R9.2 v8.89,13.46
  Bottom 0.178: v8.89,13.46 JP1.1
N$9
  Top 0.203: D1.C 8.5,24.13 8.91,24.54 10.77,24.54 11.02,24.29 U1.1
N$14
  Top 0.203: U1.5 13.62,24.35 13.17,24.8 R6.2
N$17
  Top 0.203: R3.2 5.88,24.16 D1.A
SCK  (via drill 0.25)
  Top 0.203: v14.33,40.84 14.01,41.16 U2.26
  Bottom 0.178: 17.78,40.64 14.53,40.64 v14.33,40.84
  Bottom 0.203: J2.11 20.22,39.37 19.84,39.75 18.67,39.75 17.78,40.64
SCL  (via drill 0.25)
  Top 0.178: R5.1 7.33,8.47 6.75,7.9 J3.4
  Top 0.203: U2.44 13.18,37.24 12.01,38.41 v11.61,38.41 | J3.4 3.33,7.9 v3.17,7.75
  Route15 0.203: v11.61,38.41 11.92,38.41 12.29,38.04 12.29,35.15 4.29,27.15 4.29,8.26 3.78,7.75 v3.17,7.75
  Bottom 0.203: v11.61,38.41 11.61,38.69 11.1,39.2 11.1,42.68 9.28,44.5 9.28,44.99 9.78,45.48 9.78,49.28 8.51,50.55 5.71,50.55 4.7,49.53 J1.11
SDA  (via drill 0.25)
  Top 0.152: 8.04,10.58 6.36,8.9 6.34,8.9
  Top 0.178: 6.34,8.9 J3.3 | R9.1 8.04,10.58
  Top 0.203: U2.43 12.68,37.2 12.37,37.51 11.79,37.51 v11.68,37.62 | J3.3 v3.12,8.89 | v6.48,49.91 6.48,50.67 5.08,52.07 J1.12
  Route15 0.203: v11.68,37.62 11.68,35.81 3.12,27.25 v3.12,8.89
  Bottom 0.203: v11.68,37.62 11.48,37.82 11.37,37.82 10.72,38.47 10.72,42.52 8.9,44.34 8.9,45.14 9.4,45.64 9.4,49.02 8.51,49.91 v6.48,49.91
SWDCLK
  Top 0.203: U2.57 18.54,42.16 18.91,42.53 18.91,42.54 19.05,42.68 TP2.P$1
SWDIO
  Top 0.203: U2.58 18.15,42.66 18.4,42.91 18.4,43.45 19.05,44.1 TP1.P$1
V_BATT
  Top 0.406: J1.1 3.56,24.13 4.32,23.37 4.32,19.81 4.59,19.54 J4.2 10.02,19.54 10.88,20.4 Q1.3 11.94,21.84 11.74,22.04 U1.3 9.55,22.04 C6.1
V_USB  (via drill 0.25)
  Top 0.203: R3.1 7.58,26.38 v7.62,26.42 | 13.65,22.01 14.31,22.01 14.44,21.88 C19.1
  Top 0.305: Q1.1 10.99,17.72 10.66,17.39 D2.A 10.67,16 10.16,15.49 10.16,4.66 J6.VBUS
  Top 0.406: Q1.1 10.99,19.12 11.18,19.3 13.34,19.3 13.62,19.59 U1.4 | U1.4 13.65,22.01 | v13.97,22.86 13.62,22.51 U1.4 | R7.2 C19.1
  Bottom 0.406: v13.97,22.86 13.51,22.4 8.33,22.4 7.62,23.11 v7.62,26.42 7.62,28.7 7.11,29.21 J1.3
VCC
  Top 0.203: U2.53 17.68,40.16 17.96,39.89 17.96,39.67 18.26,39.36 C13.1 19.84,40.79 19.94,40.79 C14.1
VDDA
  Top 0.203: L1.2 9.51,49.95 C12.1 10.11,49.97 10.16,49.91 10.8,49.91 10.86,49.97 C15.1 10.92,49.15 11.68,48.39 U2.8 11.68,46.87 11.94,46.61 13.46,46.61 13.68,46.83 U2.4
VIN
  Top 0.203: C7.1 15.66,26.58 15.88,26.8 15.88,27.6 15.89,27.62 15.89,28.95 14.87,29.97 R2.2
  Top 0.305: D2.C 12.96,17.52 12.89,17.59 12.89,18.29 Q1.2
  Top 0.406: 12.89,18.29 14.07,18.29 14.46,17.9 15.77,17.9 15.99,18.13 15.99,24.73 15.4,25.32 15.32,25.32 15.11,25.53 C7.1 15.09,26.61 U3.1
XIN32
  Top 0.203: U2.1 15.18,49.72 15.49,50.04 Y1.P$1 16.76,50.04 16.82,50.09 C1.1
XOUT32
  Top 0.203: U2.2 14.68,49.71 14.35,50.04 Y1.P$2 12.95,50.04 12.9,50.09 C2.1

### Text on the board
Top: 1
Route2: 2
Route15: 3
Bottom: 4 | v10
tPlace: + | -
Measures: Units in inches
tDocu: Mike Hord, Mary West & Andy England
